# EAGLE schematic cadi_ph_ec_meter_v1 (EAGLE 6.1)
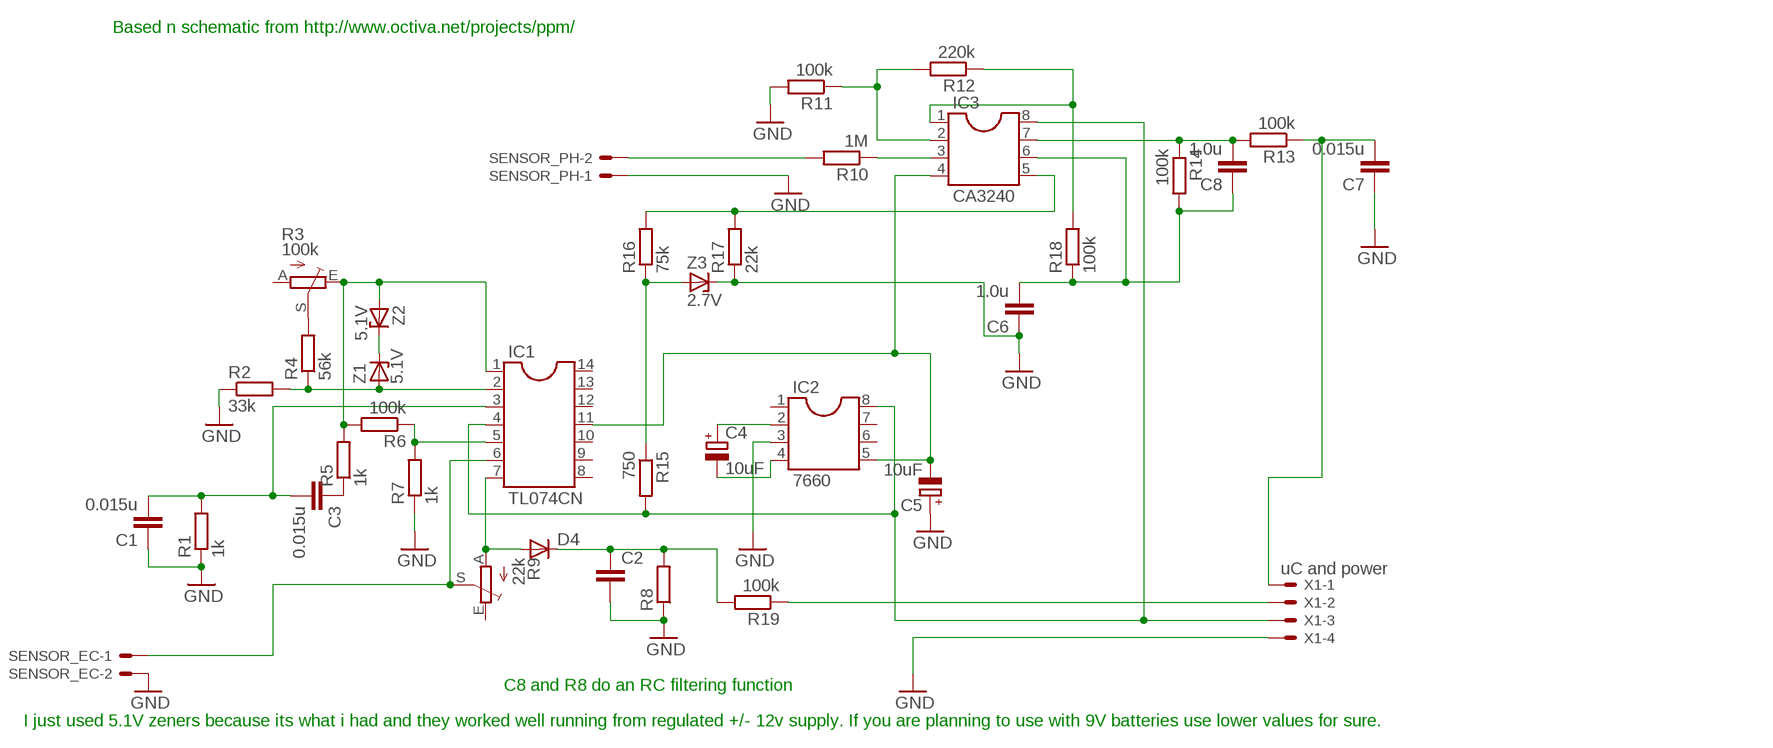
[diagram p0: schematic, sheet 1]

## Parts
C1  0.015u  C-EU050-024X044  [C050-024X044]
C2  C-EU050-045X075  [C050-045X075]
C3  0.015u  C-EU050-024X044  [C050-024X044]
C4  10uF  CPOL-EUE5-4  [E5-4]
C5  10uF  CPOL-EUE5-4  [E5-4]
C6  1.0u  C-EU050-024X044  [C050-024X044]
C7  0.015u  C-EU050-024X044  [C050-024X044]
C8  1.0u  C-EU050-024X044  [C050-024X044]
D4  BAT81  [DO34-7]
IC1  TL074CN  DIL14  [DIL14]
IC2  7660  DIL8  [DIL08]
IC3  CA3240  DIL8  [DIL08]
R1  1k  R-EU_0207/7  [0207/7]
R2  33k  R-EU_0207/7  [0207/7]
R3  100k  TRIM_EU-LI10  [LI10]
R4  56k  R-EU_0207/7  [0207/7]
R5  1k  R-EU_0207/7  [0207/7]
R6  100k  R-EU_0207/7  [0207/7]
R7  1k  R-EU_0207/7  [0207/7]
R8  R-EU_0207/7  [0207/7]
R9  22k  TRIM_EU-LI10  [LI10]
R10  1M  R-EU_0207/7  [0207/7]
R11  100k  R-EU_0207/7  [0207/7]
R12  220k  R-EU_0207/7  [0207/7]
R13  100k  R-EU_0207/7  [0207/7]
R14  100k  R-EU_0207/7  [0207/7]
R15  750  R-EU_0207/7  [0207/7]
R16  75k  R-EU_0207/7  [0207/7]
R17  22k  R-EU_0207/7  [0207/7]
R18  100k  R-EU_0207/7  [0207/7]
R19  100k  R-EU_0207/7  [0207/7]
SENSOR_EC  22-23-2021  [22-23-2021]
SENSOR_PH  22-23-2021  [22-23-2021]
X1  uC and power  22-23-2041  [22-23-2041]
Z1  5.1V  ZENER-DIODEDO34-7  [DO34Z7]
Z2  5.1V  ZENER-DIODEDO34-7  [DO34Z7]
Z3  2.7V  ZENER-DIODEDO34-7  [DO34Z7]

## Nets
GND: C1.1 C2.2 C5.+ C6.1 C7.1 IC2.3 R1.1 R2.1 R7.1 R8.1 R11.2 R17.1 SENSOR_EC.2 SENSOR_PH.1 X1.4 Z3.C
N$1: IC1.2 R2.2 R4.1 Z1.A
N$2: R3.S R4.2
N$3: IC1.1 R3.E R5.2 R6.2 Z2.A
N$4: Z1.C Z2.C
N$5: C1.2 C3.2 IC1.3 R1.2
N$6: IC1.5 R6.1 R7.2
N$7: C3.1 R5.1
N$8: D4.A IC1.7 R9.A
N$9: IC1.6 R9.S SENSOR_EC.1
N$10: C2.1 D4.C R8.2 R19.2
N$11: C5.- IC1.11 IC2.5 IC3.4
N$12: C4.+ IC2.2
N$13: C4.- IC2.4
N$14: IC3.3 R10.1
N$15: IC1.4 IC2.8 IC3.8 R15.2 X1.3
N$16: R10.2 SENSOR_PH.2
N$17: IC3.2 R11.1 R12.2
N$18: R15.1 R16.1 Z3.A
N$19: R19.1 X1.2
N$20: IC3.5 R16.2 R17.2
N$21: C6.2 C8.1 IC3.6 R14.2 R18.1
N$22: IC3.1 R12.1 R18.2
N$24: C8.2 IC3.7 R13.2 R14.1
N$26: C7.2 R13.1 X1.1
Unconnected: IC1.8 IC1.9 IC1.10 IC1.12 IC1.13 IC1.14 IC2.1 IC2.6 IC2.7 R3.A R9.E

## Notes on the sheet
- Based n schematic from http://www.octiva.net/projects/ppm/
- C8 and R8 do an RC filtering function
- I just used 5.1V zeners because its what i had and they worked well running from regulated +/- 12v supply. If you are planning to use with 9V batteries use lower values for sure.

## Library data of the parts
C1-C3 C6-C8 = resistor:C-EU: CAPACITOR, European symbol
C4 C5 = resistor:CPOL-EU: POLARIZED CAPACITOR, European symbol
D4 = diode:BAT81: DIODE
IC1 = ic-package:DIL14: Dual In Line / Socket
IC2 IC3 = ic-package:DIL8: Dual In Line / Socket
R1 R2 R4-R8 R10-R19 = resistor:R-EU_: RESISTOR, European symbol
R3 R9 = pot:TRIM_EU-: POTENTIOMETER
SENSOR_EC SENSOR_PH = con-molex:22-23-2021: .100" (2.54mm) Center Header - 2 Pin; MF: MOLEX; MPN: 22-23-2021; OC_FARNELL: 1462926; OC_NEWARK: 25C3832
X1 = con-molex:22-23-2041: .100" (2.54mm) Center Header - 4 Pin; MF: MOLEX; MPN: 22-23-2041; OC_FARNELL: 1462920; OC_NEWARK: 38C0355
Z1-Z3 = diode:ZENER-DIODE: Z-Diode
